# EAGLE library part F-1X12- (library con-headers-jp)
FEMALE HEADER
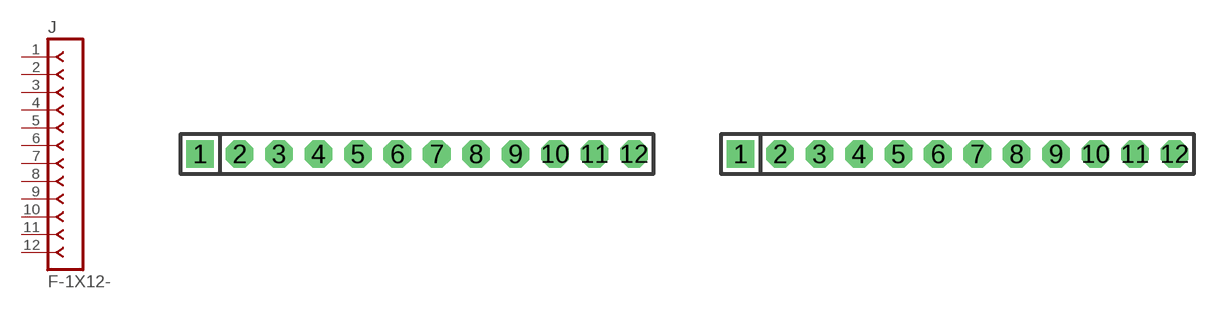
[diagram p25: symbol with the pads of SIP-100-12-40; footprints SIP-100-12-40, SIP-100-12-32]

Designator prefix J

## F-1X12-SIP-100-40  [SIP-100-12-40]
1  1  pas
2  2  pas
3  3  pas
4  4  pas
5  5  pas
6  6  pas
7  7  pas
8  8  pas
9  9  pas
10  10  pas
11  11  pas
12  12  pas

## F-1X12-SIP-100-32  [SIP-100-12-32]
Pads as for SIP-100-12-40

## F-1X12-SIP-100-32Y  [SIP-100-12-32Y]
Pads as for SIP-100-12-40

## F-1X12-SIP-100-40Y  [SIP-100-12-40Y]
Pads as for SIP-100-12-40

## F-1X12-KK-4455-B12  [KK-4455-B12]
Pads as for SIP-100-12-40

## F-1X12-KK-4455-C12  [KK-4455-C12]
Pads as for SIP-100-12-40

## F-1X12-KK-4455-A12  [KK-4455-A12]
Pads as for SIP-100-12-40

## Footprint SIP-100-12-40 (pad centres in mm)
SIP Header - 0.1", 40 mil drill
drill 1.016 pad 1.778 square: 1 -13.97,0
drill 1.016 pad 1.778 octagon: 2 -11.43,0; 3 -8.89,0; 4 -6.35,0; 5 -3.81,0; 6 -1.27,0; 7 1.27,0; 8 3.81,0; 9 6.35,0; 10 8.89,0; 11 11.43,0; 12 13.97,0

## Footprint SIP-100-12-32 (pad centres in mm)
SIP Header - 0.1", 32 mil drill
drill 0.813 pad 1.778 square: 1 -13.97,0
drill 0.813 pad 1.778 octagon: 2 -11.43,0; 3 -8.89,0; 4 -6.35,0; 5 -3.81,0; 6 -1.27,0; 7 1.27,0; 8 3.81,0; 9 6.35,0; 10 8.89,0; 11 11.43,0; 12 13.97,0

## Footprint SIP-100-12-32Y (pad centres in mm)
SIP Header - 0.1", 32 mil drill
drill 0.813 long: 1 -13.97,0; 2 -11.43,0; 3 -8.89,0; 4 -6.35,0; 5 -3.81,0; 6 -1.27,0; 7 1.27,0; 8 3.81,0; 9 6.35,0; 10 8.89,0; 11 11.43,0; 12 13.97,0

## Footprint SIP-100-12-40Y (pad centres in mm)
SIP Header - 0.1", 40 mil drill
drill 1.016 long: 1 -13.97,0; 2 -11.43,0; 3 -8.89,0; 4 -6.35,0; 5 -3.81,0; 6 -1.27,0; 7 1.27,0; 8 3.81,0; 9 6.35,0; 10 8.89,0; 11 11.43,0; 12 13.97,0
